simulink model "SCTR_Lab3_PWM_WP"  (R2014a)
settings: Solver=FixedStepDiscrete  StartTime=0.0  StopTime=inf  FixedStep=1e-6  RelTol=1e-3
libraries: simulink x1, powerlib_meascontrol x1

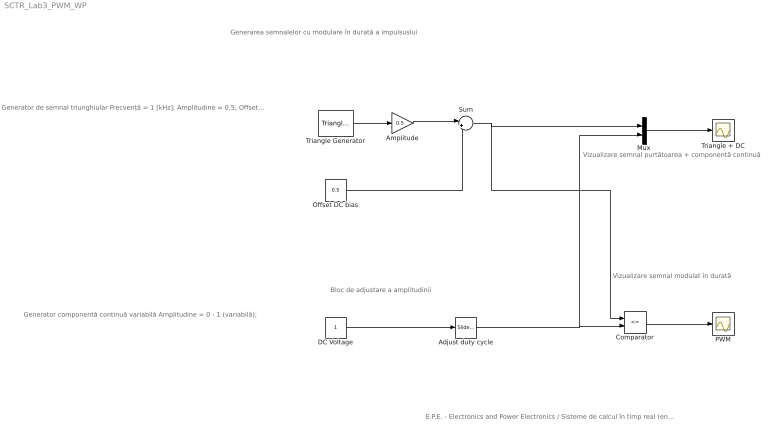
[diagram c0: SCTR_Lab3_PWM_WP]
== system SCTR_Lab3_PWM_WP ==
  note: Generator de semnal triunghiular Frecvență = 1 [kHz]; Amplitudine = 0,5; Offset = 0,5;
  note: Generarea semnalelor cu modulare în durată a impulsuslui
  note: E.P.E. - Electronics and Power Electronics / Sisteme de calcul în timp real (eng. Real - time computing systems) http://epe.utcluj.ro/index.php/sisteme-de-calcul-in-timp-real/ Subject: „Real - time computing systems” Model title: „How P.W.M. works?” Model done by: Pintilie Lucian Nicolae e-mail: Lucian.Pintilie@emd.utcluj.ro
  note: Generator componentă continuă variabilă Amplitudine = 0 - 1 (variabilă);
  note: Bloc de adjustare a amplitudinii
  note: Vizualizare semnal modulat în durată
  note: Vizualizare semnal purtătoarea + componentă continuă
  Adjust duty cycle : simulink/Math Operations/Slider Gain  low=0  gain=0  high=1
  Amplitude : Gain  Gain=0.5
  Comparator : RelationalOperator  Operator=<=  OutDataTypeStr=boolean
  DC Voltage : Constant
  Mux : Mux  Inputs=2
  Offset DC bias : Constant  Value=0.5
  PWM : Scope
  Sum : Sum  Inputs=|++
  Triangle Generator : powerlib_meascontrol/Pulse & Signal Generators/Triangle Generator  Freq=1000  Phase=0  Ts=0
  Triangle + DC : Scope
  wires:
  DC Voltage/1 -> Adjust duty cycle/1
  Adjust duty cycle/1 -> Mux/2, Comparator/2
  Comparator/1 -> PWM/1
  Mux/1 -> Triangle + DC/1
  Triangle Generator/1 -> Amplitude/1
  Sum/1 -> Mux/1, Comparator/1
  Offset DC bias/1 -> Sum/2
  Amplitude/1 -> Sum/1
